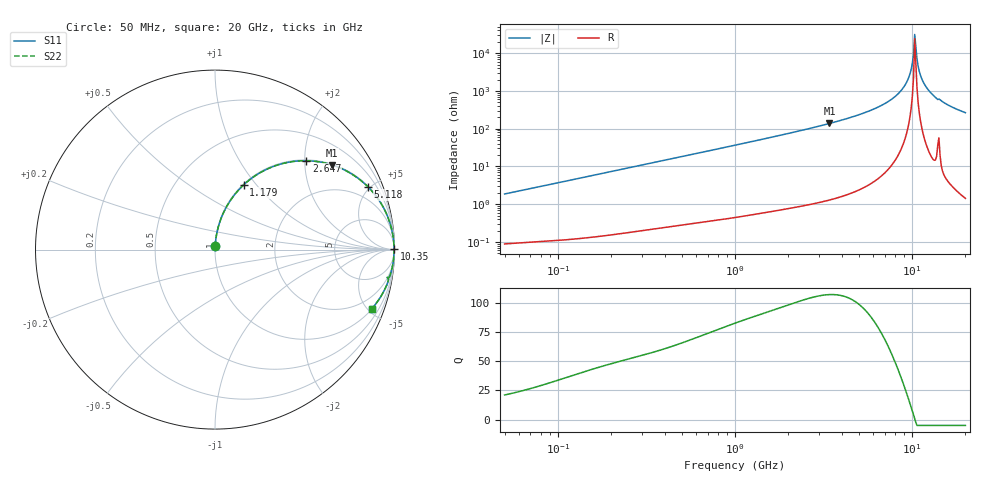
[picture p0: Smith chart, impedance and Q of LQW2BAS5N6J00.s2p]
!Murata Part Number: LQW2BAS5N6J00
!These Parameters are Measured in Series Mode Connection
!  o--[Z]--o
!Port1  Port2
!  o-------o
!Freq. Start=50[MHz] Stop=20[GHz], 401[Steps]
# Hz S RI R 50
!Freq.(Hz) S11(Real) S11(Imag) S21(Real) S21(Imag) S12(Real) S12(Imag) S22(Real) S22(Imag)
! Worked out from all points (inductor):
!   401 points, 50 MHz to 20 GHz, reference 50 ohm
!   read as one part in series: L = 5.89 nH near 51.52 MHz
!   highest Q = 107 at 3.415 GHz (marker M1), where L = 6.41 nH
!   self-resonance near 10.35 GHz
!   S11 on the Smith chart (normalised r, x): 50 MHz: 1.00, +0.04; 1.179 GHz: 1.01, +0.86; 2.647 GHz: 1.02, +2.03; 5.118 GHz: 1.05, +4.85; 10.35 GHz: open; 20 GHz: 1.03, -5.31
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5e7  0.00123 0.0186  0.9988 -0.0186  0.9988 -0.0186  0.00123 0.0186
1.364002e8  0.00374 0.0499  0.9963 -0.0499  0.9963 -0.0499  0.00374 0.0499
3.721004e8  0.0202 0.1326  0.9798 -0.1326  0.9798 -0.1326  0.0202 0.1326
1e9  0.1204 0.3194  0.8796 -0.3194  0.8796 -0.3194  0.1204 0.3194
1.179116e9  0.1597 0.3605  0.8403 -0.3605  0.8403 -0.3605  0.1597 0.3605
2.647493e9  0.5086 0.4951  0.4914 -0.4951  0.4914 -0.4951  0.5086 0.4951
2.728004e9  0.5255 0.4946  0.4745 -0.4946  0.4745 -0.4946  0.5255 0.4946
3.415248e9  0.6526 0.4715  0.3474 -0.4715  0.3474 -0.4715  0.6526 0.4715
5.117541e9  0.8519 0.3501  0.1481 -0.3501  0.1481 -0.3501  0.8519 0.3501
7.442007e9  0.965 0.1756  0.035 -0.1756  0.035 -0.1756  0.965 0.1756
8.516016e9  0.9859 0.1056  0.0141 -0.1056  0.0141 -0.1056  0.9859 0.1056
9.316812e9  0.994 0.058  0.00599 -0.058  0.00599 -0.058  0.994 0.058
9.745021e9  0.9963 0.0341  0.0037 -0.0341  0.0037 -0.0341  0.9963 0.0341
1.019291e10  0.9974 0.01  0.00259 -0.01  0.00259 -0.01  0.9974 0.01
1.034674e10  0.9975 0.002  0.00247 -0.002  0.00247 -0.002  0.9975 0.002
1.066139e10  0.9974 -0.0141  0.00263 0.0141  0.00263 0.0141  0.9974 -0.0141
1.098561e10  0.9967 -0.0301  0.00332 0.0301  0.00332 0.0301  0.9967 -0.0301
1.131968e10  0.9955 -0.0462  0.00453 0.0462  0.00453 0.0462  0.9955 -0.0462
1.257102e10  0.987 -0.1024  0.013 0.1024  0.013 0.1024  0.987 -0.1024
1.354865e10  0.9756 -0.1437  0.0244 0.1437  0.0244 0.1437  0.9756 -0.1437
1.550395e10  0.9524 -0.2077  0.0476 0.2077  0.0476 0.2077  0.9524 -0.2077
2e10  0.8746 -0.3285  0.1254 0.3285  0.1254 0.3285  0.8746 -0.3285
